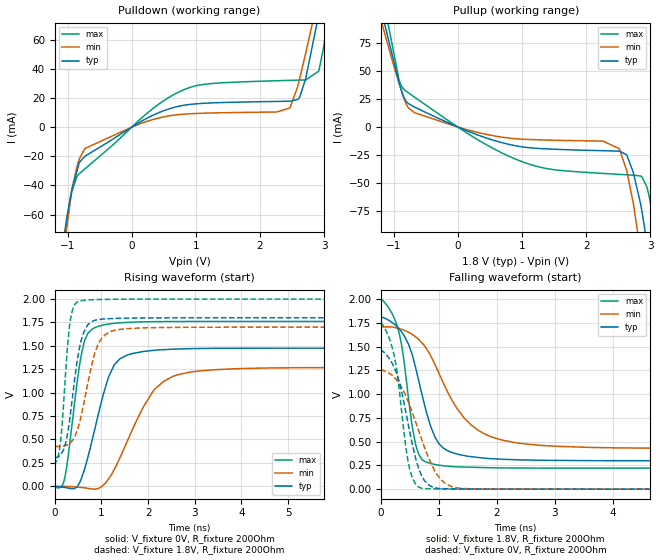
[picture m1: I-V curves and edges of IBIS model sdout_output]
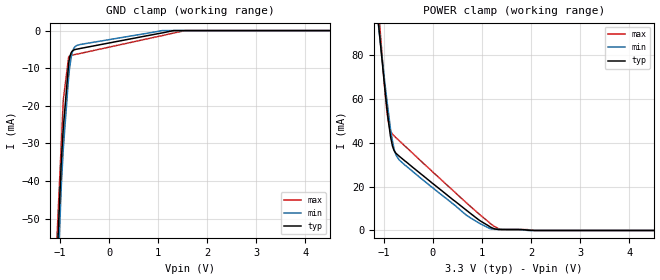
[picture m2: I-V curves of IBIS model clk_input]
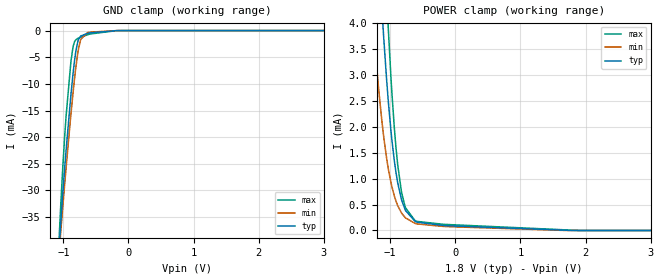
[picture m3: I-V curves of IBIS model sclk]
|Texas Instruments Incorporated
| ADS58J6x Quad-Channel, 14-Bit, 500-MSPS Telecom Receiver Device
| Marketing part#   Digital Voltage Range   Package-type   #pins
| ads58j6xI   1.1V-3.6V   QFN   72
[IBIS Ver]   4.1
[File name]   ads58j6x.ibs
[File Rev]   1.0
[Date]   4/10/2015
[Source]
| Texas Instruments Incorporated.
| Analog-eLab Design Center, HPA
| 12500 TI Blvd
| Dallas, TX -75243
[Notes]   Revision History:
| Rev 1.0: 6/26/2015
| - Initial version of the model
| - Model generated from simulations in TISPICE
| - Model matched to SPICE simulation
| - C_comp although listed in numerical order of value are
|   obtained from varying PVT conditions. For PVT conditions for
|   each specific value refer the buffer description under
|   respective [Model]. IBIS model user is responsible for using
|   appropriate C_comp to simulate for Signal Integrity.
[Disclaimer]
| This model is designed as an aid for customers of Texas Instruments.
| TI and its licensors and suppliers make no warranties, either expressed
| or implied, with respect to this  model, including the warranties of
| merchantability or fitness for a particular purpose. The model is
| provided solely on an "as is" basis. The entire risk as to its quality
| and performance is with the customer.
[Copyright]
(C) Copyright 2015 Texas Instruments Incorporated.All rights reserved.
|   ads58j6x
[Component]   ads58j6x
[Manufacturer]   TI
[Package]   |72 QFN
|   typ   min   max
R_pkg   1.09071   0.62039   1.42465
L_pkg   0.94900nH   0.49300nH   1.33000nH
C_pkg   0.11141pF   0.09250pF   0.14100pF
[Pin]  signal_name   model_name   R_pin   L_pin   C_pin
1   TRDYCD   sdout_output   1.48956   1.30000nH  0.10300pF
2   TRIGCD   syncb   1.31827   1.14000nH  0.11300pF
3   DGND   power   1.09712   0.81700nH  0.12600pF
4   IOVDD   power   1.03373   0.78300nH  0.13300pF
5   SDIN   sdio   1.19838   1.07000nH  0.11000pF
6   SCLK   sclk   1.27028   1.10000nH  0.11400pF
7   SEN   sen   1.29674   1.19000nH  0.12100pF
8   DVDD   power   1.01654   0.70900nH  0.18900pF
9   AVDD   power   1.15409   0.84800nH  0.16800pF
10   AVDD3V   power   1.31230   0.91000nH  0.17700pF
11   SDOUT   sdout_output   1.39074   1.33000nH  0.14100pF
12   AVDD   power   1.09867   0.78300nH  0.21500pF
13   INDP   nc   1.19226   0.85500nH  0.18400pF
14   INDM   nc   1.07331   0.88400nH  0.19100pF
15   AVDD   power   1.13237   0.77900nH  0.21500pF
16   AVDD3V   power   0.97876   0.74500nH  0.19000pF
17   AVDD   power   1.09275   0.75100nH  0.20600pF
18   INCM   nc   1.70877   1.36000nH  0.11300pF
19   INCP   nc   1.71115   1.25000nH  0.10800pF
20   AVDD   power   1.02981   0.91600nH  0.10600pF
21   AGND   gnd   0.73299   0.76300nH  0.09960pF
22   NC   nc   0.60486   0.47600nH  0.11100pF
23   NC   nc   0.65794   0.45600nH  0.12000pF
24   AVDD3V   power   0.66727   0.51900nH  0.11800pF
25   AVDD   power   0.65110   0.48500nH  0.11800pF
26   AGND   gnd   0.60526   0.44800nH  0.12400pF
27   CLKINP   clk_input   0.62039   0.49300nH  0.10600pF
28   CLKINM   clk_input   0.71666   0.49700nH  0.10800pF
29   AGND   gnd   0.78587   0.43300nH  0.12200pF
30   AVDD   power   0.70343   0.48300nH  0.11900pF
31   AVDD3V   power   0.70871   0.51700nH  0.12000pF
32   AGND   gnd   0.71831   0.44800nH  0.11900pF
33   SYSREFP   sysref   0.80966   0.71700nH  0.09250pF
34   SYSREFM   sysref   0.85362   0.78300nH  0.09980pF
35   AVDD   power   1.03233   0.94800nH  0.10500pF
36   INBP   nc   1.59850   1.22000nH  0.10900pF
37   INBM   nc   1.95805   1.32000nH  0.11400pF
38   AVDD   power   1.34266   0.71900nH  0.20900pF
39   AVDD3V   power   1.29753   0.70900nH  0.19100pF
40   AVDD   power   1.28059   0.72800nH  0.21700pF
41   INAM   nc   1.26582   0.84200nH  0.19300pF
42   INAP   nc   1.26182   0.80100nH  0.18400pF
43   AVDD   power   1.21899   0.74400nH  0.21700pF
44   AVDD   power   1.56735   1.24000nH  0.14200pF
45   AVDD3V   power   1.27037   0.82900nH  0.18800pF
46   AVDD   power   1.46444   0.79900nH  0.17000pF
47   DVDD   power   1.09908   0.68100nH  0.18800pF
48   RESET   reset   1.42465   1.23000nH  0.12700pF
49   SCAN_EN   scanen   1.37702   1.13000nH  0.12000pF
50   PDN   pdn   1.24691   1.04000nH  0.10400pF
51   IOVDD   power   1.13566   0.76700nH  0.13000pF
52   DGND   gnd   1.03787   0.77100nH  0.12500pF
53   TRIGAB   syncb   1.30999   1.09000nH  0.11400pF
54   TRDYAB   sdout_output   1.50259   1.25000nH  0.10400pF
55   SYNCbABP   sysref   1.94872   1.70000nH  0.16200pF
56   SYNCbABM   sysref   1.44363   1.38000nH  0.17100pF
57   IOVDD   power   0.96111   0.86300nH  0.17400pF
58   DAP   nc   1.17246   1.10000nH  0.12500pF
59   DAM   nc   0.98947   0.91300nH  0.09840pF
60   DGND   gnd   0.80726   0.60200nH  0.11900pF
61   DBP   nc   1.11795   1.03000nH  0.11100pF
62   DBM   nc   0.95457   0.85900nH  0.10400pF
63   DGND   gnd   0.94187   0.80900nH  0.10000pF
64   IOVDD   power   0.71731   0.56400nH  0.11800pF
65   DCM   nc   0.99097   0.85900nH  0.10300pF
66   DCP   nc   1.09606   1.03000nH  0.11400pF
67   DGND   gnd   0.83460   0.75200nH  0.13600pF
68   DDM   nc   1.23430   1.18000nH  0.13900pF
69   DDP   nc   1.46768   1.45000nH  0.14700pF
70   IOVDD   power   0.92410   0.90300nH  0.16900pF
71   SYNCbCDM   sysref   1.50046   1.41000nH  0.16900pF
72   SYNCbCDP   sysref   1.96842   1.73000nH  0.15800pF
[Diff_pin]   inv_pin   vdiff   tdelay_typ   tdelay_min   tdelay_max
27   28   0.2   NA   NA   NA
33   34   0.45   NA   NA   NA
55   56   0.45   NA   NA   NA
72   71   0.45   NA   NA   NA
| Models and submodels in the file (10): sdout_output (Output), clk_input (Input), sclk (Input), sen (Input), syncb (Input), scanen (Input), sdio (I/O), sysref (Input), pdn (Input), reset (Input)
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|   SDOUT_OUTPUT Model
[Model]   sdout_output
Model_type   Output
Polarity   Non-Inverting
Vmeas = 0.9
Vref = 0
Cref = 1pF
Rref = 10000
|   typ   min   max
C_comp   0.533pF   0.488pF   0.563pF
| Where nom  PVT is Nominal Process, 1.8V, 25C
|   Fast PVT is Strong Process,  2.0V, -40C
|   Slow PVT is Weak Process,   1.7V, 85C
[Voltage Range]   1.8   1.7   2
[Temperature Range]   25   85   -40
[Pullup Reference]   1.8   1.7   2
[Pulldown Reference]   0   0   0
[Power Clamp Reference]   1.8   1.7   2
[GND Clamp Reference]   0   0   0
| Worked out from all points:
|   slope of the pulldown table from 0 to 0.27 V, typ, clamps not added: 39.4 ohm
|   slope of the pullup table from 0 to 0.27 V, typ, clamps not added: 43.3 ohm
|   falling waveform, V_fixture 1.8V, R_fixture 200Ohm: 20-80 % time 407ps typ, 724ps min, 252ps max; typ from 1.8 V to 0.299 V
|   rising waveform, V_fixture 0V, R_fixture 200Ohm: 20-80 % time 462ps typ, 758ps min, 276ps max; typ from 0 V to 1.48 V
|   rising waveform, V_fixture 1.8V, R_fixture 200Ohm: 20-80 % time 253ps typ, 342ps min, 158ps max; typ from 0.299 V to 1.8 V
|   falling waveform, V_fixture 0V, R_fixture 200Ohm: 20-80 % time 322ps typ, 473ps min, 225ps max; typ from 1.48 V to 0 V
[Pulldown]
|   Voltage   I(typ)   I(min)   I(max)
-1.8V     -414.3mA   -413.1mA   -419.5mA
-1.022V   -64.87mA   -72mA      -68.67mA
-936mV    -43.44mA   -43.16mA   -44.59mA
-817.2mV  -24.16mA   -21.72mA   -31.9mA
-730.8mV  -19.95mA   -14.64mA   -28.65mA
597.6mV   12.75mA    7.848mA    20.85mA
2.466V    17.79mA    13.16mA    32.09mA
2.617V    20.52mA    33.1mA     32.28mA
2.714V    33.87mA    51.22mA    32.4mA
2.914V    77.04mA    90.5mA     38.35mA
3.044V    106.2mA    117.5mA    69.14mA
3.584V    237mA      235.1mA    225.1mA
[Pullup]
|   Voltage   I(typ)   I(min)   I(max)
-1.8V     245.5mA    219.1mA    301.7mA
-1.001V   59mA       54.73mA    66.43mA
-882mV    32.63mA    32.53mA    36.74mA
-676.8mV  17.89mA    12.87mA    26.78mA
921.6mV   -16.88mA   -10.47mA   -29.13mA
2.261V    -21.05mA   -12.47mA   -41.36mA
2.52V     -21.49mA   -19.91mA   -42.24mA
2.633V    -25.18mA   -39.75mA   -42.61mA
2.844V    -67.91mA   -110.8mA   -43.67mA
2.941V    -101.8mA   -153.3mA   -52.93mA
3.087V    -165.6mA   -220.4mA   -91.53mA
3.584V    -406mA     -450.9mA   -314.3mA
[Ramp]
R_load = 200
|   typ   min   max
dV/dt_r   0.885158/4.61781e-10   0.760591/7.56151e-10   1.05665/2.75743e-10
dV/dt_f   0.900469/4.06737e-10   0.762816/7.19365e-10   1.06711/2.49394e-10
[Falling Waveform]
V_fixture = 1.8V
V_fixture_min = 1.7V
V_fixture_max = 2V
R_fixture = 200Ohm
|   Time   V(typ)   V(min)   V(max)
0s        1.8V       1.7V       2V
294.3ps   1.7V       1.694V     1.684V
381.4ps   1.632V     1.678V     1.414V
475.3ps   1.525V     1.652V     947.2mV
598.4ps   1.275V     1.603V     467.4mV
787.6ps   800.3mV    1.475V     283.7mV
1.076ns   431.2mV    1.116V     246.4mV
1.538ns   343.6mV    684.6mV    231.3mV
2.125ns   314mV      511.7mV    223.7mV
7.552ns   299.2mV    428.6mV    221.5mV
[Rising Waveform]
V_fixture = 0V
V_fixture_min = 0V
V_fixture_max = 0V
R_fixture = 200Ohm
|   Time   V(typ)   V(min)   V(max)
0s        -70.99nV   -315.6nV   16.4nV
215.5ps   -12.73mV   -1.299mV   92.27mV
478.2ps   -4.249mV   -8.249mV   1.106V
639.4ps   184.7mV    -16.75mV   1.558V
852.5ps   600.2mV    -30.55mV   1.693V
1.152ns   1.167V     78.17mV    1.733V
1.4ns     1.363V     308.3mV    1.746V
2.1ns     1.451V     1.01V      1.758V
2.531ns   1.465V     1.173V     1.76V
7.328ns   1.475V     1.268V     1.761V
[Rising Waveform]
V_fixture = 1.8V
V_fixture_min = 1.7V
V_fixture_max = 2V
R_fixture = 200Ohm
|   Time   V(typ)   V(min)   V(max)
0s        299.2mV    428.7mV    221.5mV
70.83ps   316.2mV    425mV      314.4mV
136.6ps   344.3mV    426.3mV    534.4mV
251.9ps   495.8mV    439mV      1.359V
317.2ps   699mV      458.5mV    1.718V
485.6ps   1.356V     604.5mV    1.972V
628ps     1.654V     897.6mV    1.987V
865.7ps   1.774V     1.436V     1.994V
1.218ns   1.792V     1.658V     1.998V
7.328ns   1.8V       1.7V       2V
[Falling Waveform]
V_fixture = 0V
V_fixture_min = 0V
V_fixture_max = 0V
R_fixture = 200Ohm
|   Time   V(typ)   V(min)   V(max)
0s        1.475V     1.268V     1.761V
196.1ps   1.322V     1.197V     1.484V
315.5ps   1.128V     1.114V     1.042V
411.3ps   863.6mV    1.006V     521.4mV
488.5ps   624.2mV    889.7mV    224.5mV
653.2ps   209.5mV    607.1mV    20.23mV
787.6ps   63.1mV     381.1mV    5.3mV
949.9ps   11.71mV    169.8mV    2.788mV
1.305ns   3.059mV    14.17mV    648.5uV
7.552ns   -299.1nV   -1.086uV   -289.1nV
|   CLK_INPUT Model
[Model]   clk_input
Model_type   Input
Vinl = 0.6
Vinh = 1.4
|   typ   min   max
C_comp   0.783pF   0.664pF   1.069pF
| Where nom  PVT is Nominal Process, 3.3V, 25C
|   Fast PVT is Strong Process,  3.6V, -40C
|   Slow PVT is Weak Process,   3.0V, 85C
[Voltage Range]   3.3   3   3.6
[Temperature Range]   25   85   -40
[Power Clamp Reference]   3.3   3   3.6
[GND Clamp Reference]   0   0   0
[GND Clamp]
|   Voltage   I(typ)   I(min)   I(max)
-3.3V     -930mA     -923mA     -939mA
-1.11V    -75.9mA    -86.1mA    -68.3mA
-974mV    -34.5mA    -40.9mA    -29.66mA
-934mV    -25.8mA    -31.3mA    -18.3mA
-825mV    -8.7mA     -12.2mA    -6.99mA
-776mV    -5.95mA    -7.26mA    -6.61mA
-746mV    -5.39mA    -5.56mA    -6.51mA
-706mV    -5.1mA     -4.45mA    -6.39mA
-647mV    -4.91mA    -3.9mA     -6.23mA
1.07V     -646uA     -20.7uA    -1.37mA
1.54V     0A         0A         -10.5uA
6.6V      0A         0A         0A
[POWER Clamp]
|   Voltage   I(typ)   I(min)   I(max)
-3.3V     512mA      455mA      631mA
-1.42V    165mA      156mA      191mA
-993mV    67.92mA    70.22mA    67.6mA
-914mV    51.3mA     55.1mA     50.2mA
-865mV    43mA       46.6mA     45.4mA
-825mV    38.6mA     40.9mA     44mA
-736mV    34.9mA     33.8mA     42mA
670mV     9.46mA     7.19mA     12.9mA
1.17V     1.56mA     832uA      3.15mA
1.4V      415uA      493uA      455uA
2.07V     0A         0A         0A
6.6V      0A         0A         0A
|   sclk Model
[Model]   sclk
Model_type   Input
Vinl = 0.4
Vinh = 1.2
|   typ   min   max
|   (nom PVT)   (fast PVT)   (slow PVT)
|Average
C_comp   1.163e-12   1.143e-12   1.183e-12
| Where nom  PVT is Nominal Process, 1.8V, 25C
|   Fast PVT is Strong Process,  1.9V, -40C
|   Slow PVT is Weak Process,   1.7V, 85C
[Voltage Range]   1.8   1.7   1.9
|Ambient Temperature   25   85   -40
|Junction Temperature
[Temperature Range]   25   85   -40
[Power Clamp Reference]   1.8   1.7   1.9
[GND Clamp Reference]   0   0   0
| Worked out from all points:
|   GND clamp passes 1 mA (typ) near -0.73 V on its own axis
|   POWER clamp passes 1 mA (typ) near -0.90 V on its own axis
[GND Clamp]
|   Voltage   I(typ)   I(min)   I(max)
-1.8V     -253.9mA   -233.1mA   -272.1mA
-1.072V   -42.59mA   -42.97mA   -41.16mA
-1.057V   -39.51mA   -40.55mA   -37.19mA
-1.039V   -35.98mA   -37.69mA   -32.62mA
-958.3mV  -22.65mA   -25.91mA   -16.25mA
-882.3mV  -11.96mA   -15.62mA   -5.724mA
-848.1mV  -7.815mA   -11.39mA   -2.936mA
-806.4mV  -3.809mA   -6.82mA    -1.712mA
-732.2mV  -1.014mA   -1.647mA   -1.25mA
-630.4mV  -542.4uA   -390.4uA   -803.9uA
-180mV    -8.61uA    -7.386uA   -10.29uA
3.6V      0A         0A         0A
[POWER Clamp]
|   Voltage   I(typ)   I(min)   I(max)
-1.8V     24.9mA     16.77mA    34.61mA
-1.251V   7.237mA    3.849mA    11.04mA
-1.173V   5.291mA    2.673mA    8.221mA
-1.101V   3.759mA    1.827mA    5.905mA
-1.028V   2.483mA    1.186mA    3.878mA
-973.8mV  1.747mA    844.2uA    2.657mA
-935.5mV  1.337mA    662.1uA    1.967mA
-884.2mV  918.9uA    479.8uA    1.265mA
-829.1mV  610.6uA    344.9uA    768.4uA
-763.2mV  383.2uA    241.7uA    435.2uA
-618.5mV  177.2uA    136.5uA    190.3uA
3.6V      0A         0A         0A
